FUNCTION_BLOCK "DRVHandling"
TITLE =SERVOSTAR
//V2.0
//Datum    : 06.01.2004
//Name     : J.Schellhorn
//Homepage : www.DanaherMotion.net
AUTHOR : JSCHN
NAME : SSTR
VERSION : 2.0


VAR_INPUT
  BUS_Address : INT  := 3;	//Node-Address of Profibus / Profibus-Teilnehmer-Adresse
  NUDB : INT  := 100;	//No. of User-DataBlock / Nummer des Nutzdatenbausteins
  PERI_Address : INT  := 8;	//Periphery - address defined in hardware(PKW)/Peripherie adresse wie Hardware
  SW_Enable : BOOL ;	//Drive enable (Software-Enable) / Freigabe Servo (Software)
  Reset_Fault : BOOL ;	//Reset Fault / Reset Fehler
  Jog_for : BOOL ;	//Jog + / Tippen +
  Jog_back : BOOL ;	//Jog - / Tippen -
  Ref_Start : BOOL ;	//Start reference move / Start Referenzfahrt
  Start_MT : BOOL ;	//Motion Task MT / Start Fahrsatz
  Fast_Stop_Disable : BOOL ;	//Fast-Stop with disable drive / Not-Halt mit Einschaltsperre
  Fast_Stop_Enable : BOOL ;	//Fast-Stop without disabling drive / Not-Halt ohne Einschaltsperre
  Pause : BOOL ;	//Pause in Motion Task / Unterbrechung von Fahraufträgen
  Position_Reset : BOOL ;	//Reset position / Rücksetzen der Position
  Accept_Values : BOOL ;	//Accept new values / Neue Werte übernehmen
  Init_Drive : BOOL ;	//Initalize drive / Initialisierung des Reglers
END_VAR
VAR_OUTPUT
  Actual_Speed : WORD ;	//Actual speed / Istdrehzahl
  Actual_Position : DWORD ;	//Actual position / Istposition
  Manufac_Stat : WORD ;	//Manufacturer Status / Herstellerstatus
  ZSW : WORD ;	//Status word of axis / Zustandsword der Achse
  Error : BOOL ;	//Error-bit / Sammelfehlerbit
  Pos_Error : BOOL ;	//Warning Pos.error / Warnung Schleppfehler angesprochen
  Moving : BOOL ;	//Motor is moving / Motor dreht
  Reference_ok : BOOL ;	//Reference ok / Referenz vorhanden
  In_Position : BOOL ;	//In position / Antrieb ist in Position
  ACK_ready_ok : BOOL ;	//Acknowledge operation ready without fault / Angeforderte Aktion fertig
  ACK_ready_fault : BOOL ;	//Acknowledge operation ready with fault Angeforderte Aktion fertig mit Fehler
  MT_active : BOOL ;	//Motion Task active / Fahrsatz aktiv
END_VAR
VAR
  nudbnr : WORD ;
  NUDB_Adr : WORD ;
  conv_stw : WORD ;
  conv_stat : WORD ;
  conv_zsw : WORD ;
  conv_akku1 : DWORD ;
  kfeh : BOOL ;
  busy : BOOL ;
  ofeh : BOOL ;
  mfeh : BOOL ;
  send : BOOL ;
  redy : BOOL ;
  status : WORD ;
  parameter_nr : WORD ;
  parameter_index : BYTE ;
  read_write_flag : BOOL ;
  start_flag : BOOL ;
  aktiv : BOOL ;
  fertig : BOOL ;
  fehler : BOOL ;
  ref_ok : BOOL ;
  parametertyp : BYTE ;
  parameter_high : WORD ;
  parameter_low : WORD ;
  reset_flag : BOOL ;
  pf_ref_start : BOOL ;
  ref_art_ok : BOOL ;
  ba_ok : BOOL ;
  enable_ok : BOOL ;
  init_ok : BOOL ;
  null_ok : BOOL ;
  sypa : INT ;
  modus : INT  := 2;	//Modus
  FlankeP : BOOL ;	// Bitmerker für positive Flanke
  FlankeN : BOOL ;	// Bitmerker für negative Flanke
  FlaMemP : BOOL ;	// Bitmerker für positive Flanke
  FlaMemN : BOOL ;	// Bitmerker für positive Flanke
  FlaP_RI : BOOL ;	// Bitmerker für positive Flanke
  FlaMemP_RI : BOOL ;	// Bitmerker für positive Flanke
  Init_Drive_Flag : BOOL ;	//Flag for Initalization Drive
  Accept_Values_Flag : BOOL ;	//Flag to accept new values
  Bit_Step : ARRAY  [1 .. 16 ] OF //Status Bits
  BOOL ;
  TaccOK : BOOL ;	//Beschleunigungszeitwert übernommen
  TdecOK : BOOL ;	//Verzögerungszeitwert übernommen
  PNU_OK : BOOL ;	//PNU und Parameter übernommen
  ZERO_OK : BOOL ;	//Nulltelegramm geschrieben
  NrKSTW : WORD ;
  PKWReceive : ARRAY  [1 .. 8 ] OF BYTE ;
  PZDReceive : ARRAY  [1 .. 12 ] OF BYTE ;
  PKWSend : ARRAY  [1 .. 4 ] OF WORD ;
  PZDSend : ARRAY  [1 .. 6 ] OF WORD ;
  PKWPeriStart : WORD ;
  PZDPeriStart : WORD ;
  ErgPZD : INT ;
  ErgPKW : INT ;
  SendPKW : INT ;
  Empf : INT ;
  Stop_MT : BOOL ;
  pf_flag_ref : BOOL ;
  pf_flag_values : BOOL ;
  Accept_flag : BOOL ;
  te1 : WORD ;
  te2 : WORD ;
END_VAR
VAR_TEMP
  conv_nudb : WORD ;
END_VAR
BEGIN
NETWORK
TITLE =Preset adresses User data block (NUDB)

      L     #NUDB;
      T     #NUDB_Adr;

      L     0;
      T     #NrKSTW;


      L     #PERI_Address; // startaddress PKW in periphery
      T     #PKWPeriStart;

      L     #PERI_Address;
      L     8;
      +I    ;
      T     #PZDPeriStart; // startaddress PZD in periphery

NETWORK
TITLE =Select function Reset Fault and Warnings

      L     #NUDB_Adr;
      T     #conv_nudb;
      AUF   DB [#conv_nudb]; // UserData DB

      U     #Reset_Fault; //Reset errors , warnings
      =     DBX   27.7;
      U     #Reset_Fault;
      U     DBX   47.7; // error / fault
      =     DBX   26.5; // Warning
NETWORK
TITLE =Set Message Outputs
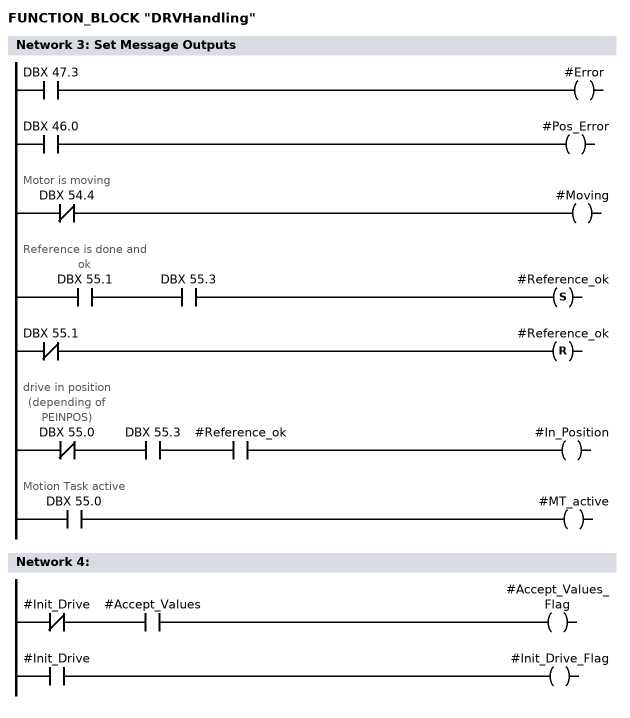
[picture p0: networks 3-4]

      O     DBX   47.3;
      =     #Error;

      U     DBX   46.0;
      =     #Pos_Error;

      UN    DBX   54.4; // Motor is moving
      =     #Moving;

      U     DBX   55.1; // Reference is done and ok
      U     DBX   55.3;
      S     #Reference_ok;
      UN    DBX   55.1;
      R     #Reference_ok;

      UN    DBX   55.0; // drive in position (depending of PEINPOS)
      U     DBX   55.3;
      U     #Reference_ok;
      =     #In_Position;

      U     DBX   55.0; // Motion Task active
      =     #MT_active;


NETWORK
TITLE =

      UN    #Init_Drive;
      U     #Accept_Values;
      =     #Accept_Values_Flag;

      U     #Init_Drive;
      =     #Init_Drive_Flag;


NETWORK
TITLE =Initialisierung (Nulltelegramm)

      U     #Init_Drive_Flag;
      UN    #FlaMemP_RI;
      =     #FlaP_RI;
      U     #FlaP_RI;
      S     #FlaMemP_RI;
      UN    #Init_Drive_Flag;
      R     #FlaMemP_RI;

      U     #ba_ok;
      UN    #Init_Drive_Flag;
      R     #Bit_Step[5];
      R     #Bit_Step[6];

      U     #Bit_Step[5];
      U     #fehler;
      R     #Bit_Step[5];

      U     #Bit_Step[5];
      U     #fertig;
      UN    #aktiv;
      S     #Bit_Step[6];
      R     #Bit_Step[5];

      U     #Bit_Step[4];
      UN    #fertig;
      U     #aktiv;
      S     #Bit_Step[5];
      R     #Bit_Step[4];

      U     #Bit_Step[3];
      UN    #fertig;
      UN    #aktiv;
      S     #Bit_Step[4];
      R     #Bit_Step[3];

      U     #Bit_Step[2];
      UN    #aktiv;
      U     #fertig;
      S     #Bit_Step[3];
      R     #Bit_Step[2];

      U     #Bit_Step[1];
      U     #aktiv;
      UN    #fertig;
      S     #Bit_Step[2];
      R     #Bit_Step[1];

      U     #Init_Drive_Flag; //Reset bei Fehlern und Anlauf
      UN    #ba_ok;
      UN    #Bit_Step[1];
      UN    #Bit_Step[2];
      UN    #Bit_Step[3];
      UN    #Bit_Step[4];
      UN    #Bit_Step[5];
      UN    #Bit_Step[6];
      S     #Bit_Step[1];

      U     #FlaP_RI;
      R     #Bit_Step[1];
      R     #Bit_Step[2];
      R     #Bit_Step[3];
      R     #Bit_Step[4];
      R     #Bit_Step[5];
      R     #Bit_Step[6];
      R     #fertig;
      R     #start_flag;
      R     #read_write_flag;
      R     #ba_ok;
      R     DBX   26.2;
      UN    #FlaP_RI;
      SPB   M001;
      L     0;
      T     DBD   18;
      T     DBD   22;
      T     DBD   26;
      T     DBD   30;
      T     DBD   34;

M001: NOP   0;

      U     #fehler;
      R     #start_flag;
      R     #read_write_flag;

      UN    #Bit_Step[1];
      UN    #Bit_Step[2];
      UN    #Bit_Step[3];
      SPB   M002;
      L     3;
      T     #parametertyp;

M002: NOP   0;

      U     #Bit_Step[1];
      S     #read_write_flag;
      S     #start_flag;

      U     #Bit_Step[3];
      R     #start_flag;
      R     #read_write_flag;

      UN    #Bit_Step[4];
      UN    #Bit_Step[5];
      UN    #Bit_Step[6];
      SPB   M003;

      L     2;
      T     #parametertyp;

      L     W#16#3A2;
      T     #parameter_nr;

      L     DBW   80;
      T     #parameter_low;

      L     DBW   80;

      L     0;
      <I    ;
      SPB   M054;

      L     0;
      SPA   M055;
M054: NOP   0;
      L     W#16#FFFF;


M055: NOP   0;
      T     #parameter_high;
M003: NOP   0;
      U     #Bit_Step[4];
      S     #read_write_flag;
      S     #start_flag;
      U     #Bit_Step[6];
      R     #start_flag;
      R     #read_write_flag;
      S     #ba_ok;
NETWORK
TITLE =Setting Values for ACC and DCC and PNU
//Write Parameter with PNU declared in DBNU.DBW  84 and the belonging value in
//DBNU.DBD  86.
      U     #Accept_Values_Flag;
      UN    #pf_flag_values;
      =     #Accept_flag;
      S     #pf_flag_values;

      UN    #Accept_Values_Flag;
      R     #pf_flag_values;

      UN    #Accept_Values_Flag;
      R     #PNU_OK;
      R     #ZERO_OK;

      UN    #Accept_flag;
      SPB   M004;

      U     #PNU_OK;
      SPB   M004;

      U     #ZERO_OK;
      SPB   M005;

      L     0;
      T     DBW   18;

      U(    ;
      L     DBW   38;
      L     0;
      ==I   ;
      )     ;
      U     #Accept_Values_Flag;
      UN    #PNU_OK;
      S     #ZERO_OK;

M005: NOP   0;

      UN    #ZERO_OK;
      SPB   M004;

      L     2;
      T     #parametertyp;

      L     W#16#1;
      T     #parameter_index;

      L     DBW   84; //Betriebsartenumschaltung ??
      L     W#16#3A2; //PNU930
      <>I   ;
      SPB   M006;
      L     DBW   84;
      T     #parameter_nr;
      U     DBX   26.2; // PZD sperren (Bit 10 im STW)
      R     DBX   26.2;
      SPA   M007;

M006: NOP   0;

      UN    DBX   83.2;
      SPB   M008;
      L     DBW   84;
      T     #parameter_nr;
      SPA   M009;

M008: NOP   0;

      L     DBW   84;
      +     1600;
      T     #parameter_nr;

M009: NOP   0;

      L     #parameter_nr;
      L     2047;
      <=I   ;
      SPB   M007;
      L     #parameter_nr;
      +     -400;
      T     #parameter_nr;

      L     W#16#11;
      T     #parameter_index;

M007: NOP   0;

      U     #Accept_flag;
      U     DBX   83.1;
      S     #read_write_flag;

      U     #Accept_flag;
      UN    DBX   83.1;
      R     #read_write_flag;

      UN    #read_write_flag;
      SPB   M010;

      L     DBW   86;
      T     #parameter_high;

      L     DBW   88;
      T     #parameter_low;

      SPA   M011;

M010: NOP   0;

      L     DBW   42;
      T     DBW   76;

      L     DBW   44;
      T     DBW   78;

M011: NOP   0;
      U     #Accept_Values_Flag;
      S     #start_flag;

      U     #ZERO_OK;
      U     #fertig;
      U     #Accept_Values_Flag;
      S     #PNU_OK;
      R     #start_flag;
      R     #ZERO_OK;

      NOP   0;


      UN    #PNU_OK;
      SPB   M004;
//
      L     3;
      T     #parametertyp;

      UN    #ZERO_OK;
      S     #read_write_flag;

      U     #fertig;
      U     #Accept_Values_Flag;
      U     #PNU_OK;
      S     #ZERO_OK;
      R     #start_flag;
      S     DBX   26.2;

      UN    #fertig;
      U     #Accept_Values_Flag;
      U     #PNU_OK;
      S     #start_flag;
      S     DBX   26.2; // PZD freigeben (Bit10 im STW)

M004: NOP   0;

      U     #Bit_Step[6];
      U     #Init_Drive_Flag;
      O     ;
      U     #PNU_OK;
      U     #ZERO_OK;
      UN    #fehler;
      =     #ACK_ready_ok;
//      S     DBX   26.2

      U     #fehler;
      U(    ;
      O     #PNU_OK;
      O     #ZERO_OK;
      )     ;
      O(    ;
      U     DBX   38.4;
      U     DBX   38.6;
      U(    ;
      O     #Accept_Values;
      O     #Init_Drive;
      )     ;
      )     ;
      =     #ACK_ready_fault;


NETWORK
TITLE =Betriebsartenanwahl

      U     #SW_Enable;
      U     #ba_ok;
      =     DBX   27.0;
      =     DBX   27.1;

      U     DBX   47.0;
      U     DBX   47.1;
      U     #SW_Enable;
      =     DBX   27.3;

      U     #ba_ok;
      U     DBX   27.0; // STW Bit0 : Einschalten
      U     DBX   27.3; // STW Bit3 : Betrieb freigeben
      U     DBX   47.2;
      SPB   M012;

      ON    #SW_Enable;
      ON    #ba_ok;
      SPB   M013;

      U     #ba_ok;
      U     DBX   27.0; // STW Bit0 : Einschalten
      U     DBX   27.3; // STW Bit3 : Betrieb freigeben
      SPB   M012;

M013: NOP   0;

      UN    #SW_Enable;
      R     #enable_ok;

      L     DBW   38;
      SRW   12;
      L     B#16#7;
      ==I   ;
      R     #init_ok;

      SPA   M014;

M012: NOP   0;


NETWORK
TITLE =Antrieb enablen

      U     #enable_ok;
      SPB   M015;

      L     DBW   26;
      L     W#16#43F; //Enablen des Servostar (Hardwareenable muss anstehen !!!)
      OW    ;
      T     DBW   26; // STW beschreiben

      U     DBX   47.0;
      U     DBX   47.1;
      U     DBX   47.5;
      UN    DBX   47.6;
      S     #enable_ok;

      ON    #SW_Enable;
      O     DBX   47.6;
      R     #enable_ok;




      U     #enable_ok;
      SPB   M015;

      UN    #enable_ok;
      R     DBX   27.3;

      SPA   M014;

M015: NOP   0;

NETWORK
TITLE =Tippbetrieb

      UN    #Jog_for; //Tippen vorwärts angewählt
      UN    #Jog_back;
      O     ;
      U     #Jog_for;
      U     #Jog_back;
      SPB   M016;

      U     #Jog_back; //Tippen rückwärts angewählt
      SPB   M017;
      L     DBW   58; //Tippgeschwindigkeit (für vorwärts positiv)
      T     DBW   28;
      SPB   M016;
M017: NOP   0;
      L     DBW   58; //Tippgeschwindigkeit
      L     -1; //(für rückwärts negativ)
      *I    ;
      T     DBW   28;
M016: NOP   0;
      U     #Jog_for; //Tippgeschwindigkeit auf Null und Steuerbit reset
      UN    #Jog_back;
      O     ;
      UN    #Jog_for;
      U     #Jog_back;
      =     DBX   26.0;
      R     #Stop_MT;
NETWORK
TITLE =Referenzfahrt

      ON    #Ref_Start;
      O     #ref_ok;
      SPB   M014;

      L     DBW   60;
      T     DBW   28;

      L     W#16#C3F;
      T     DBW   26;

      UN    DBX   55.0;
      U     DBX   55.3;
      U     DBX   55.1;
      S     #ref_ok;


M014: NOP   0;
      UN    #Ref_Start; // Abbruch Referenzfahrt
      R     DBX   26.3; // reset Start Referenzfahrt

      UN    #Ref_Start;
      UN    DBX   55.1;
      R     #ref_ok;

      U     #Fast_Stop_Disable;
      =     DBX   27.2;

      U     #Fast_Stop_Enable;
      =     DBX   27.4;

      UN    #Pause;
      =     DBX   27.5;


      U     #Position_Reset;
      =     DBX   26.4;

      L     DBW   26;
      T     #conv_stw;

      U     #Ref_Start;
      FP    #pf_ref_start;
      =     #pf_flag_values;
      U     #pf_flag_values;
      R     #ref_ok;
      R     #Stop_MT;
NETWORK
TITLE =
//alter FC106/FB106 / Fahrsatz aufrufen und abarbeiten
      L     2;
      T     #modus;
NETWORK
TITLE =Gesamtnetzwerk
// Fahrsatz starten
      U(    ;
      L     #modus;
      L     2;
      <>I   ; // Betriebsart = Positionierung?
      )     ;
      ON    DBX   55.1;
      ON    #Reference_ok;
      O     DBX   26.0;
      O     #Ref_Start;
      SPB   M018; // Nein, dann nicht bearbeiten

      UN    #Start_MT; // Bit zum Starten eines Fahrauftrages
      U     #FlaMemN; // negativer Flankenmerker
      =     #FlankeN;
      R     #FlaMemN;

      U     #Start_MT;
      S     #FlaMemN;


      U     #Start_MT; // Bit zum Starten eines Fahrsatzes
      UN    #FlaMemP; // Flankenmerker
      =     #FlankeP;
      S     #FlaMemP;

      UN    #Start_MT;
      R     #FlaMemP;

      U     #FlankeN;
      U     DBX   83.0; // Vorwahl mit Toggeln
      SPB   M019; // Bei Flanke Fahrauftrag beenden

      U     #FlankeN;
      UN    DBX   83.0;
      SPB   M020;

      U     #FlankeP;
      SPB   M021;

      SPA   M022; // zum Ausgang

M020: NOP   0; // Zeiger auf Steuerwort
      U     #FlankeN;
      S     #Stop_MT;

      SPA   M022;

M019: NOP   0;
      U     DBX   27.6; // Bit 6 im STW
      R     DBX   27.6;

      SPA   M022;

M021: NOP   0; //

      U     #Stop_MT;
      R     #Stop_MT;

      UN    DBX   83.0;
      U     DBX   27.6;
      R     DBX   27.6;
      SPB   M022;

      UN    DBX   27.6; // Abfrage Bit 6 im STW
      S     DBX   27.6; // Sollwertfreigabe / Start Fahrsatz

M022: NOP   0;




      L     DBW   62;
      L     0;
      <>I   ; // Fahrsatznummer ungleich 0
      SPB   M023; // dann gespeicherten Fahrsatz starten
      NOP   0; // Programmteil für Direktfahraufträge
      UN    DBX   26.6; // Lade Steuerwort
      S     DBX   26.6; // Bit 14 = 1 (PZD - Direktfahrsatz)


      UN    DBX   27.3; // Bit 3 setzen und Betrieb freigeben
      S     DBX   27.3;

      L     DBD   66; // Sollgeschwindigkeit
      T     DBD   28; // in Peripherie schreiben

      L     DBD   70; // Sollposition
      T     DBD   32; // in Peripherie schreiben

      L     DBW   64; // Fahrsatzart
      T     DBW   36; // in Peripherie schreiben
      SPA   M018;

M023: NOP   0; // Programmteil für gespeicherte Fahraufträge, STW Bit14=0
      U     DBX   26.6; // Lade Steuerwort
      R     DBX   26.6; // Bit 14 = 0  (PZD (HSW) - Fahrsatznummer)

      UN    DBX   27.3; // Bit 3 setzen und Betrieb freigeben
      S     DBX   27.3;


      L     DBW   62;
      T     DBW   28; // im Prozeßdatenbereich ablegen

M018: NOP   0;
      U     #Stop_MT;
      R     DBX   27.3;


NETWORK
TITLE =
//alter FC110/FB110 Transfer von Parametern, Ist- und Sollwerten zwischen
//Steuerung und
//Antrieb
      L     #NUDB_Adr;
      T     #conv_nudb;
      AUF   DB [#conv_nudb]; // Nutzdaten DB


      U     #start_flag;
      SPB   M024; // liegt an

      L     DW#16#0;
      T     DBW    0;

      U     M      0.0;
      ON    M      0.0; // immer 1
      R     #fertig; // alles zuruecksetzen
      R     #aktiv;
      R     #fehler;

      L     #status;
      L     W#16#FF7F;
      UW    ; // Status korrigieren (alt R M 239.7)
      T     #status;

      SPA   M025; // -> Ende
M024: U     #fehler;
      O     #fertig; // wenn fertig nicht nochmal lesen
      SPB   M026;
      UN    #read_write_flag; // Parameter lesen
      SPB   M027;
      SPA   M028; // Bei S7 direkter Sprung möglich, 16.5.1997
M027: NOP   0; // alt: U     M    239.7 // Laeuft Parameteraktion
      L     #status;
      L     W#16#80;
      UW    ;
      L     128;
      ==I   ;
      SPB   M029; // Parameter lesen
      O     DBX    5.0; // PKW-Auftrag laeuft
      SPB   M025; // Zwischenstation zum Ende
      S     #aktiv;

      L     #status;
      L     W#16#180; // S M 239.7   //Parameteraktion starten
      OW    ; // S M 238.0   //Busy
      T     #status;
      L     W#16#1000; // PKE/AK = 1 (lesen)
      L     #parameter_nr; // Parameternummer
      OW    ; // verknuepfen
      T     #conv_akku1;
      L     #conv_akku1;
      T     DBW   18; // PKE schreiben
// neu: 7.2.2000, Aufnahme des Index
      L     #parameter_index;
      SLW   8;
      T     #conv_akku1;

      L     DBW   20; // IND lesen
      L     W#16#FF;
      UW    ;
      L     #conv_akku1;
      OW    ;
      T     DBW   20; // IND schreiben, bis hier: 7.2.2000

//      L     W#16#1                      // PKW-Auftrag starten : Parameter lesen
//      T     #conv_akku1

//      L     #conv_akku1
//      T     DBW   20                    // abspeichern

M025: L     #status; //MW   238
      T     #status;
      SPA   M026;
      SPA   M030; // Zwischenstation zum Para-
      NOP   0; // meter schreiben
M029: NOP   0; // Ist Parameter schon da?
      NOP   0; // PKE im Empfangsfach, PPO-Typ2
      L     DBW   38;
      L     W#16#7FF;
      UW    ; // PNU extrahieren
      L     #parameter_nr; // =abgeschickter Parameternr.?
      <>I   ;
      SPB   M025; // nein -> Status speichern, Rücksprung zum Ende
      NOP   0; // neu: 7.2.2000, Abfrage des Index
      NOP   0; // IND lesen vorbereiten
      L     DBW   40;
      SRW   8; // 10.2.2000
      L     #parameter_index; // =abgeschicktem Index?
      <>I   ;
      SPB   M025; // nein -> Status speichern, Rücksprung zum Ende
      L     DBW   38; // Überprüfung der Antwort, Wort/Doppelwort/generell OK
      L     W#16#F000;
      UW    ; // AK ausblenden
      L     W#16#7000; // Parameterauftrag fehlerhaft ?
      ==I   ;
      SPB   M031; // Ja !
      SPA   M032; // Nein !
M031: S     #fehler; // sonst Fehlerbit setzen
      L     W#16#FFFF;
      T     #parameter_high; // High-Wort Parameter ungültig
      NOP   0; // PWE2 im Empfangsfach
      L     DBW   44; // holen
      T     #parameter_low; // Fehlernummer im Parameter-Low-Wort
      SPA   M025; // und beenden
M032: NOP   0;
      L     DBW   38; // Überprüfung der Antwort, Wort/Doppelwort/generell OK
      SRW   12; // oberstes Nibble nach unten holen
      T     #parametertyp; // PTYP zuweisen
      L     2; // Doppelwortparameter ?
      ==I   ;
      SPB   M033; // Ja !
      L     0; // Bei Wortparametern High-Wort immer auf 0 setzen
      T     #parameter_high;
      SPA   M034; // Low-Wort aus DP-Fach holen
M033: NOP   0;
      L     DBW   42; // PWE1 lesen
      T     #parameter_high; // ausgeben
M034: NOP   0;
      L     DBW   44; // PWE2 lesen
      T     #parameter_low; // ausgeben
      SPA   M035; // Sprungmarke ueberspringen
M030: SPA   M028;
M035: SPB   M036; // Fertig, VKE immer "1"
M036: S     #fertig; // Fertigbit setzen
      R     #aktiv; // Aktivbit zuruecknehmen
      R     #fehler; // Fehlerbit loeschen

      L     #status;
      L     W#16#FE7F;
      UW    ; // Status korrigieren (alt R M 239.7 / R M 238.0)
      T     #status;

      SPA   M026; // Statuswort abspeichern
M028: NOP   0;
NETWORK
TITLE =

      L     #status; //      U     M    239.7   // laeuft Parameteraktion?
      L     W#16#80;
      UW    ;
      L     128;
      ==I   ;
      SPB   M037; // ja, dann Antwort pruefen
      S     #aktiv;

      L     #status;
      L     W#16#180;
      OW    ; // Status korrigieren (alt S M 239.7 / S M 238.0)
      T     #status;


      L     #parametertyp; // Typ des Parameters
      L     1; // 1 = Wort, 2 = Doppelwort
      ==I   ;
      SPB   M038; // nur ein Wort lesen, AK = 2
      L     #parametertyp;
      L     2;
      ==I   ;
      SPB   M039; // Doppelwort lesen, AK = 3
      L     #parametertyp; // 7.5.99 bei PTYP = 3 Nulltelegramm erzeugen
      L     3; // 7.5.99
      ==I   ; // 7.5.99
      SPB   M040; // 7.5.99
      S     #fehler; // sonst mit VKE = 1 Fehler setzen
      R     #aktiv; // Aktivflag zurücksetzen

      L     #status;
      L     W#16#FE7F;
      UW    ; // Status korrigieren (alt R M 239.7 / R M 238.0)
      T     #status;
      SPA   M026;
M038: NOP   0;
      L     W#16#2000; // PKE im Sendefach, AK = 2
      SPA   M041;
M040: NOP   0; // 7.5.1999 PKE und PANR auf 0
      L     W#16#0; // 7.5.1999
      SPA   M042; // 7.5.1999
M039: NOP   0;
      L     W#16#3000; // PKE im Sendefach, AK = 3
M041: L     #parameter_nr;
      OW    ; // PKE/AK (schreiben)
      NOP   0; // mit Parameternummer
M042: T     #conv_akku1;

      L     #conv_akku1;
      T     DBW   18; // PKE ins DP-Fach eintragen
      NOP   0; // neu: 7.2.2000, IND auch verarbeiten
      L     #parametertyp; // Nulltelegramm beachten, 21.2.2000
      L     3;
      <>I   ;
      SPB   M043; // Normalfall
      L     0;
      T     #conv_akku1; // 0 als Wert laden
      SPA   M044;
M043: L     #parameter_index;
      SLW   8;
      T     #conv_akku1;
      L     DBW   20; // IND lesen
      L     W#16#FF;
      UW    ;
      L     #conv_akku1;
      OW    ;
M044: T     DBW   20; // IND schreiben, bis hier: 7.2.2000

      L     #parametertyp; // Doppelwort schreiben ?
      L     2;
      ==I   ;
      SPB   M045;
      L     0; // sonst High-Wort auf 0 setzen, gilt auch für PTYP 3
      SPB   M046;
M045: L     #parameter_high; // PWE1 im Sendefach
M046: T     #conv_akku1;

      L     #conv_akku1;
      T     DBW   22; // ins DP-Sendefach eintragen

      L     #parametertyp; // 7.5.1999 bei PTYP = 3 auch PALO mit 0 schreiben
      L     3;
      <>I   ;
      SPB   M047;
      L     0; // 7.5.1999 0 laden für PTYP 3
      SPA   M048;
M047: L     #parameter_low; // PWE2 im Sendefach
M048: T     #conv_akku1;

      L     #conv_akku1;
      T     DBW   24; // Low-Wert des Parameters
      L     2#1; // Start Servoantriebsdaten
      NOP   0; // = Kommunikationsteuerwort
      T     #conv_akku1;

      L     #conv_akku1;
      T     DBW    0; // PKW-Auftrag starten
      L     #status;
      T     #status;
      SPA   M026;
M037: NOP   0;
NETWORK
TITLE =

      L     #parametertyp; // 9.5.1999 PTYP = 3 (Nulltelegramm)?
      L     3;
      <>I   ;
      SPB   M049; // 9.5.1999 PTYP 1,2, dann weiter

      L     DBW   38; // 9.5.1999, PKE, PNU lesen
      L     0;
      <>I   ;
      SPB   M026;
      U     DBX    5.4; // 9.5.1999, wenn Kommunikation gestört, Fehlerbit setzen
      SPB   M050;
      SPA   M051; // 9.5.1999, Nulltelegramm erfolgreich geschrieben
M049: NOP   0;
      L     DBW   38; // PKE lesen
      L     W#16#7FF;
      UW    ; // PNU ausblenden
      L     #parameter_nr; // mit Parameternummer
      <>I   ; // vergleichen
      SPB   M026; // wenn ungleich, dann warten
      NOP   0; // neu: 7.2.2000, auch Index vergleichen
      NOP   0; // IND lesen vorbereiten
      L     DBW   40;
      SRW   8; // 10.2.2000
      L     #parameter_index; // =abgeschicktem Index?
      <>I   ;
      SPB   M026; // wenn ungleich, dann warten
      L     #parametertyp; // Antwort typabhängig auswerten
      L     1;
      ==I   ;
      SPB   M052; // Bei Wortschreiben mit Antwort-AK 1 vergleichen
      NOP   0; // sonst mit Antwort-AK 2
      L     DBW   38; // PKE lesen
      L     W#16#F000;
      UW    ; // PKE lesen
      L     W#16#2000;
      ==I   ; // AK ausblenden
      SPB   M051; // Parameterauftrag O.K.?
      SPA   M050;
M052: NOP   0;
      L     DBW   38; // PKE lesen
      L     W#16#F000;
      UW    ; // AK ausblenden
      L     W#16#1000;
      ==I   ; // Parameterauftrag O.K.?
      SPB   M051;
M050: S     #fehler; // Fehlerbit setzen (VKE = 1)
      L     W#16#FFFF;
      T     #parameter_high; // 16.6.97, High-Wort Parameter ungültig
      L     DBW   44;
      T     #parameter_low; // 16.6.97, Fehlernummer im Parameter-Low-Wort
      SPA   M026; // und beenden
M051: S     #fertig;
      R     #aktiv; // Fehlerbit setzen

      L     #status;
      L     W#16#FE7F;
      UW    ; // Status korrigieren
      T     #status;

M026: L     #status;
      T     #status;

      L     DBW   48; // aktuelle Drehzahl holen
      T     #Actual_Speed;

      L     DBD   50; // aktuelle Position holen
      T     #Actual_Position;

      L     DBW   54; // herstellerspezifischer Status
      T     #Manufac_Stat;

      L     DBW   46;
      T     #ZSW; // ZSW

      U     DBX   83.1;
      SPB   M053;

      L     DBW   42;
      T     DBW   76;

      L     DBW   44;
      T     DBW   78;

M053: NOP   0;

NETWORK
TITLE =Receive consis. data from Profibus DP
//
//
//
// PKW - Bereich, 8 Bytes
      CALL "DPRD_DAT" (// DPRD_DAT
           LADDR                    := #PKWPeriStart,// projektierte Startadresse in Peripherie
           RET_VAL                  := #ErgPKW,// Ergebnis des Lesens
           RECORD                   := #PKWReceive);

// PZD - Bereich, 12 Bytes
      CALL "DPRD_DAT" (// DPRD_DAT
           LADDR                    := #PZDPeriStart,// projektierte Startadresse in Peripherie, PZD
           RET_VAL                  := #ErgPZD,// Ergebnis des Lesens
           RECORD                   := #PZDReceive);

NETWORK
TITLE =Write received data (PKW) to datablock (NUDB)
//
// Daten wurden gelesen, nun koennen sie in den NUDB eingetragen werden
//
      L     #NrKSTW;
      +     38;
      T     #Empf; // Start der empfangenen PKW-Daten im Nutzdatenbaustein

      SLW   3; // Zeiger auf dieses Datenwort bilden
      LAR1  ; // Adreßregister 1 laden
      L     #PKWReceive[1];
      SLW   8;
      L     #PKWReceive[2];
      OW    ; // PKW-Bereich, erstes Wort

      T     DBW [AR1,P#0.0]; // im NUDB speichern

      TAR1  ;
      +     16;
      LAR1  ;
      L     #PKWReceive[3];
      SLW   8;
      L     #PKWReceive[4];
      OW    ; // PKW-Bereich, zweites Wort

      T     DBW [AR1,P#0.0]; // im NUDB speichern

      TAR1  ;
      +     16;
      LAR1  ;
      L     #PKWReceive[5];
      SLW   8;
      L     #PKWReceive[6];
      OW    ; // PKW-Bereich, drittes Wort

      T     DBW [AR1,P#0.0]; // im NUDB speichern

      TAR1  ;
      +     16;
      LAR1  ;
      L     #PKWReceive[7];
      SLW   8;
      L     #PKWReceive[8];
      OW    ; // PKW-Bereich, viertes Wort

      T     DBW [AR1,P#0.0]; // im NUDB speichern, PKW komplett
NETWORK
TITLE =Write received data (PZD) to datablock (NUDB)
//
// PKW-Daten eingetragen, nun PZD-Daten
//
      L     #Empf;
      +     8;
      T     #Empf; // Start der empfangenen PZD-Daten im Nutzdatenbaustein

      SLW   3; // Zeiger auf dieses Datenwort bilden
      LAR1  ; // Adreßregister 1 laden
      L     #PZDReceive[1];
      SLW   8;
      L     #PZDReceive[2];
      OW    ; // PZD-Bereich, erstes Wort

      T     DBW [AR1,P#0.0]; // im NUDB speichern

      TAR1  ;
      +     16;
      LAR1  ;
      L     #PZDReceive[3];
      SLW   8;
      L     #PZDReceive[4];
      OW    ; // PZD-Bereich, zweites Wort

      T     DBW [AR1,P#0.0]; // im NUDB speichern

      TAR1  ;
      +     16;
      LAR1  ;
      L     #PZDReceive[5];
      SLW   8;
      L     #PZDReceive[6];
      OW    ; // PZD-Bereich, drittes Wort

      T     DBW [AR1,P#0.0]; // im NUDB speichern

      TAR1  ;
      +     16;
      LAR1  ;
      L     #PZDReceive[7];
      SLW   8;
      L     #PZDReceive[8];
      OW    ; // PZD-Bereich, viertes Wort

      T     DBW [AR1,P#0.0]; // im NUDB speichern

      TAR1  ;
      +     16;
      LAR1  ;
      L     #PZDReceive[9];
      SLW   8;
      L     #PZDReceive[10];
      OW    ; // PZD-Bereich, fuenftes Wort

      T     DBW [AR1,P#0.0]; // im NUDB speichern

      TAR1  ;
      +     16;
      LAR1  ;
      L     #PZDReceive[11];
      SLW   8;
      L     #PZDReceive[12];
      OW    ; // PZD-Bereich, sechstes Wort

      T     DBW [AR1,P#0.0]; // im NUDB speichern, PZD komplett
NETWORK
TITLE =Send consist. data (PKW) from datablock (NUDB) to Profibus DP
//
// PKW-Daten aus dem NUDB holen und in Felder eintragen
//
      L     #NrKSTW;
      +     18;
      T     #SendPKW; // Startadresse des PKW-Sendebereichs im Nutzdatenbaustein

      SLW   3; // Zeiger auf dieses Datenwort bilden
      LAR1  ; // Adreßregister 1 laden

      L     DBW [AR1,P#0.0]; // aus NUDB holen
      T     #PKWSend[1]; // PKW erstes Wort geladen

      TAR1  ;
      +     16;
      LAR1  ;

      L     DBW [AR1,P#0.0]; // aus NUDB holen
      T     #PKWSend[2]; // PKW zweites Wort geladen

      TAR1  ;
      +     16;
      LAR1  ;

      L     DBW [AR1,P#0.0]; // aus NUDB holen
      T     #PKWSend[3]; // PKW drittes Wort geladen

      TAR1  ;
      +     16;
      LAR1  ;

      L     DBW [AR1,P#0.0]; // aus NUDB holen
      T     #PKWSend[4]; // PKW viertes Wort geladen

      CALL "DPWR_DAT" (// DPWR_DAT
           LADDR                    := #PKWPeriStart,
           RECORD                   := #PKWSend,
           RET_VAL                  := #ErgPKW);// PKW gesendet

NETWORK
TITLE =Send consist. data (PZD) from datablock (NUDB) to Profibus DP
//
// PZD-Daten aus dem NUDB holen und in Felder eintragen
//
      L     #SendPKW;
      +     8;
      T     #SendPKW; // Startadresse des PZD - Sendebereichs im Nutzdatenbaustein

      SLW   3; // Zeiger auf dieses Datenwort bilden
      LAR1  ; // Adreßregister 1 laden

      L     DBW [AR1,P#0.0]; // aus NUDB holen
      T     #PZDSend[1]; // PZD erstes Wort geladen

      TAR1  ;
      +     16;
      LAR1  ;

      L     DBW [AR1,P#0.0]; // aus NUDB holen
      T     #PZDSend[2]; // PZD zweites Wort geladen

      TAR1  ;
      +     16;
      LAR1  ;

      L     DBW [AR1,P#0.0]; // aus NUDB holen
      T     #PZDSend[3]; // PZD drittes Wort geladen

      TAR1  ;
      +     16;
      LAR1  ;

      L     DBW [AR1,P#0.0]; // aus NUDB holen
      T     #PZDSend[4]; // PZD viertes Wort geladen

      TAR1  ;
      +     16;
      LAR1  ;

      L     DBW [AR1,P#0.0]; // aus NUDB holen
      T     #PZDSend[5]; // PZD fuenftes Wort geladen

      TAR1  ;
      +     16;
      LAR1  ;

      L     DBW [AR1,P#0.0]; // aus NUDB holen
      T     #PZDSend[6]; // PZD sechstes Wort geladen

      CALL "DPWR_DAT" (// DPWR_DAT
           LADDR                    := #PZDPeriStart,
           RECORD                   := #PZDSend,
           RET_VAL                  := #ErgPZD);// PZD gesendet

END_FUNCTION_BLOCK

